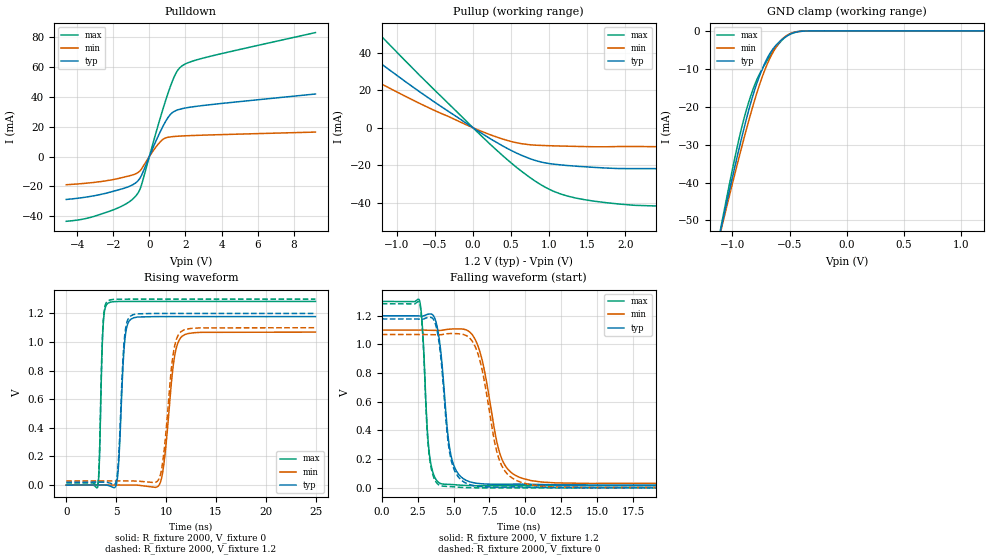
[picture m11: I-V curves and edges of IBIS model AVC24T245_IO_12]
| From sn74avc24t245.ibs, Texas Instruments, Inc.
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[Model]   AVC24T245_IO_12
Model_type  I/O
Vinl=0.385
Vinh=0.845
Enable   Active-Low
Vref =   0
Rref =   2000
Cref =   15p
Vmeas =   0.6
| variable   typ   min   max
C_comp   5.29pF   4.66pF   5.83pF
| C_pullup   5.78pF   3.89pF   7.84pF
| C_pulldown   5.32pF   4.76pF   7.02pF
| C_tri-state   5.29pF   4.66pF   5.83pF
[Temperature Range]   40   100   -40
| Ambient temperature   25   85   -40
[Voltage range]   1.2   1.1   1.3
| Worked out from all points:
|   slope of the pulldown table from 0 to 0.18 V, typ, clamps not added: 34.6 ohm
|   slope of the pullup table from 0 to 0.18 V, typ, clamps not added: 38.6 ohm
|   GND clamp passes 1 mA (typ) near -0.50 V on its own axis
|   rising waveform, R_fixture 2000, V_fixture 0: 20-80 % time 467ps typ, 865ps min, 282ps max; typ from 0 V to 1.18 V
|   falling waveform, R_fixture 2000, V_fixture 1.2: 20-80 % time 670ps typ, 1.21ns min, 399ps max; typ from 1.2 V to 0.02 V
|   rising waveform, R_fixture 2000, V_fixture 1.2: 20-80 % time 461ps typ, 848ps min, 280ps max; typ from 0.02 V to 1.2 V
|   falling waveform, R_fixture 2000, V_fixture 0: 20-80 % time 668ps typ, 1.21ns min, 397ps max; typ from 1.18 V to 0 V
[GND Clamp]
| AVC24T245_IO_12
|   Voltage   I(typ)   I(min)   I(max)
-4.6V     -597.8mA   -546.6mA   -662.5mA
-1.095V   -51.41mA   -51.9mA    -50.81mA
-1.07V    -47.97mA   -48.78mA   -46.93mA
-940mV    -30.76mA   -33.04mA   -28.1mA
-840mV    -18.99mA   -21.8mA    -17.13mA
-775mV    -12.84mA   -15.28mA   -12.1mA
-695mV    -7.204mA   -8.735mA   -7.744mA
-615mV    -3.665mA   -4.111mA   -4.191mA
-545mV    -1.809mA   -1.649mA   -1.862mA
-465mV    -549.4uA   -452.3uA   -430.6uA
-360mV    -50.53uA   -51.18uA   -21.62uA
1.2V      708.7pA    34.3nA     62.33pA
[Pulldown]
| AVC24T245_IO_12
|   Voltage   I(typ)   I(min)   I(max)
-4.6V     -28.79mA   -18.92mA   -43.46mA
-3.415V   -27.06mA   -17.81mA   -41.32mA
-2.03V    -23.44mA   -15.52mA   -35.94mA
-1.165V   -20.28mA   -13.12mA   -30.82mA
-680mV    -16.87mA   -11.13mA   -25.38mA
-435mV    -12.68mA   -8.327mA   -19.06mA
440mV     12.38mA    7.543mA    19.04mA
955mV     24.67mA    12.69mA    39.57mA
1.42V     30.53mA    13.49mA    54.64mA
1.79V     32.04mA    13.78mA    60.61mA
3.17V     34.51mA    14.41mA    66.63mA
9.2V      41.96mA    16.4mA     83.17mA
[Pullup]
| AVC24T245_IO_12
|   Voltage   I(typ)   I(min)   I(max)
-4.6V     40.24mA    7.956mA    186.3mA
-4.08V    45.4mA     8.808mA    167.8mA
-3.73V    53.62mA    9.647mA    154.2mA
-2.685V   79.31mA    16.98mA    111.4mA
-2.57V    75.87mA    21.96mA    106.5mA
-2.565V   75.72mA    49.42mA    106.3mA
-1.845V   53.66mA    37.03mA    75.82mA
-1.36V    38.76mA    26.71mA    55.3mA
575mV     -13.51mA   -7.977mA   -21.19mA
1.01V     -19.08mA   -9.527mA   -32.92mA
1.455V    -20.71mA   -9.971mA   -38.21mA
9.2V      -28.28mA   -12.48mA   -52.65mA
[Ramp]
| AVC24T245_IO_12
| variable   typ   min   max
dV/dt_r   0.72/4.81E-10   0.65/8.80E-10   0.78/2.90E-10
dV/dt_f   0.72/6.78E-10   0.65/1.22E-09   0.78/4.10E-10
R_load = 2000
[Rising Waveform]
| AVC24T245_IO_12
R_fixture =   2000
C_fixture =   0
L_fixture =   0
V_fixture =   0
V_fixture_min = 0
V_fixture_max = 0
|   Time   V(typ)   V(min)   V(max)
0s        18.11nV    102nV      416.8pV
3.155ns   608uV      -113.6uV   -13.91mV
3.685ns   448.6uV    152uV      1.099V
4.185ns   -2.315mV   116.3uV    1.272V
5.11ns    36.54mV    467.9uV    1.283V
5.825ns   978mV      363.3uV    1.284V
6.47ns    1.159V     284.2uV    1.284V
9.455ns   1.178V     21.92mV    1.284V
11.63ns   1.178V     1.041V     1.284V
24.99ns   1.178V     1.069V     1.284V
[Falling Waveform]
| AVC24T245_IO_12
R_fixture =   2000
C_fixture =   0
L_fixture =   0
V_fixture =   1.2
V_fixture_min = 1.1
V_fixture_max = 1.3
|   Time   V(typ)   V(min)   V(max)
0s        1.2V       1.1V       1.3V
2.635ns   1.198V     1.1V       1.304V
3.295ns   1.212V     1.099V     254.1mV
4.025ns   1.02V      1.098V     33.47mV
4.79ns    241mV      1.107V     23.68mV
5.885ns   51.88mV    1.102V     16.64mV
6.9ns     29mV       925.9mV    14.78mV
8.26ns    25mV       228mV      14.53mV
9.31ns    25.92mV    87mV       14.51mV
24.99ns   20.14mV    29.61mV    14.5mV
[Rising Waveform]
| AVC24T245_IO_12
R_fixture =   2000
C_fixture =   0
L_fixture =   0
V_fixture =   1.2
V_fixture_min = 1.1
V_fixture_max = 1.3
|   Time   V(typ)   V(min)   V(max)
0s        20.14mV    28.74mV    14.5mV
3.155ns   20.71mV    28.68mV    2.144mV
3.675ns   20.47mV    28.94mV    1.112V
4.14ns    18.33mV    28.87mV    1.286V
5.08ns    51.94mV    29.12mV    1.299V
5.8ns     1.001V     28.89mV    1.3V
6.425ns   1.181V     28.73mV    1.3V
9.375ns   1.2V       55.93mV    1.3V
11.51ns   1.2V       1.073V     1.3V
24.99ns   1.2V       1.1V       1.3V
[Falling Waveform]
| AVC24T245_IO_12
R_fixture =   2000
C_fixture =   0
L_fixture =   0
V_fixture =   0
V_fixture_min = 0
V_fixture_max = 0
|   Time   V(typ)   V(min)   V(max)
0s        1.178V     1.069V     1.284V
2.635ns   1.177V     1.069V     1.287V
3.29ns    1.189V     1.068V     239.3mV
4.01ns    998.8mV    1.068V     18.68mV
4.77ns    222.5mV    1.076V     8.88mV
5.885ns   31.84mV    1.062V     1.802mV
6.83ns    9.537mV    888.9mV    266.9uV
8.145ns   4.991mV    205.8mV    30.88uV
9.23ns    5.824mV    59.27mV    11.23uV
24.99ns   826.7nV    686.6uV    24.39nV
